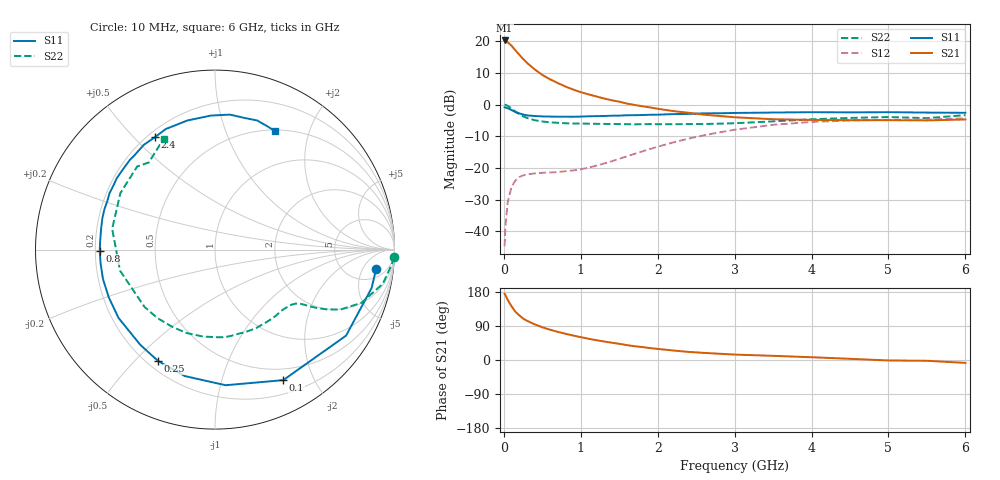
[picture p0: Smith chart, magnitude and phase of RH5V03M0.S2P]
! SIEMENS Small Signal Semiconductors
! BFR106
! Si NPN RF Bipolar Junction Transistor in SOT23
! VCE = 5 V  IC = 3 mA
! Common Emitter S-Parameters:  August  1996
# GHz  S  MA  R  50
!  f  S11  S21  S12  S22
! GHz  MAG  ANG  MAG  ANG  MAG  ANG  MAG  ANG
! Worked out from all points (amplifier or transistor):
!   36 points, 10 MHz to 6 GHz, reference 50 ohm
!   highest |S21| = 20.2 dB at 10 MHz (marker M1)
!   |S21| within 3 dB of that: start of sweep to 146.1 MHz
!   unconditionally stable (mu >= 1): 716.5 MHz to 1.87 GHz; 4.379 GHz to end of sweep
!   at 250 MHz: K = 0.39, MSG = 18.4 dB, |S12| = -22.4 dB
!   at 1.4 GHz: K = 1.18, MAG = 7.1 dB, |S12| = -17.9 dB
!   at 6 GHz: K = 1.02, MAG = -1.1 dB, |S12| = -4.4 dB
!   S11 on the Smith chart (normalised r, x): 10 MHz: 8, -10; 100 MHz: 0.36, -1.59; 250 MHz: 0.24, -0.58; 800 MHz: 0.22, -0.01; 2.4 GHz: 0.23, +0.58; 6 GHz: 0.52, +1.50
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0.01  0.9039 -7.0  10.27 175.0  0.0058 88.8  0.9974 -2.4
0.02  0.8985 -13.8  10.2 171.5  0.0117 85.4  0.9885 -4.8
0.05  0.8735 -33.3  9.616 158.5  0.0285 72.8  0.9544 -11.5
0.1  0.8207 -62.4  8.479 141.8  0.05 59.3  0.8679 -20.0
0.15  0.758 -85.5  7.176 127.4  0.0631 48.2  0.7753 -25.5
0.2  0.7244 -103.4  6.126 117.9  0.0715 42.1  0.7075 -28.1
0.25  0.6967 -117.2  5.25 109.5  0.076 37.3  0.6513 -29.9
0.3  0.6742 -128.2  4.558 103.6  0.0786 35.1  0.6137 -30.9
0.4  0.6587 -144.7  3.59 94.2  0.0817 32.5  0.5653 -32.3
0.5  0.6489 -155.8  2.931 86.3  0.0835 32.5  0.5396 -33.9
0.6  0.6453 -165.4  2.505 80.0  0.0846 34.1  0.5237 -36.0
0.8  0.6424 -179.3  1.925 69.3  0.0884 40.4  0.5058 -41.3
1.1  0.6514 164.4  1.447 56.1  0.1005 52.5  0.498 -51.0
1.6  0.6765 144.0  1.035 39.3  0.1521 66.0  0.4895 -70.4
2.2  0.7057 124.2  0.788 25.1  0.2517 65.8  0.4889 -98.0
2.4  0.7102 118.0  0.741 21.4  0.2894 63.1  0.4911 -109.0
3.5  0.7471 91.7  0.586 11.0  0.4783 40.6  0.5417 -167.4
4  0.7567 83.7  0.571 7.3  0.5309 29.2  0.5846 168.6
4.5  0.7518 77.5  0.566 3.1  0.5587 19.0  0.6138 149.2
5  0.7569 71.9  0.566 -1.2  0.5737 10.5  0.6344 133.1
5.5  0.7461 66.8  0.561 -2.1  0.5787 6.3  0.6095 127.2
6  0.7398 63.1  0.581 -7.6  0.606 -1.8  0.6801 114.9
